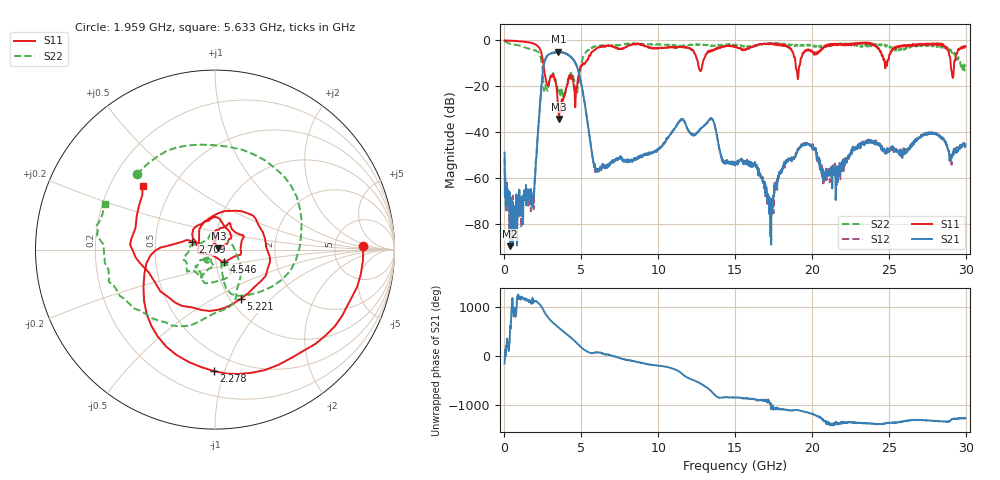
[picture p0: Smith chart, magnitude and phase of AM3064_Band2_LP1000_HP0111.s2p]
# Hz S DB R 50.0
!freq dBS11 angS11 dBS21 angS21 dBS12 angS12 dBS22 angS22
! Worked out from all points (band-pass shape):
!   1600 points, 10 MHz to 29.98 GHz, reference 50 ohm
!   highest |S21| = -4.93 dB at 3.515 GHz (marker M1); lowest = -89.5 dB at 366.1 MHz (marker M2)
!   |S21| within 3 dB of the highest: 2.68 GHz to 4.434 GHz (1.754 GHz wide, 49.3 % of centre)
!   lowest |S11| = -34.2 dB at 3.553 GHz (marker M3), VSWR 1.04, Z = 51.9 + j0.654 ohm
!   |S11| at or under -10 dB: 2.532 GHz to 5.14 GHz (2.608 GHz wide, 68 % of centre); 12.59 GHz to 12.89 GHz (294.3 MHz wide, 2.31 % of centre); 18.93 GHz to 19.24 GHz (302.5 MHz wide, 1.58 % of centre)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
!   |S22| runs from -24.7 to -0.2 dB; largest |S21 - S12| = 0.013
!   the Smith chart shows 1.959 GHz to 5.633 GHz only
!   S11 on the Smith chart (normalised r, x): 1.959 GHz: 10, +1; 2.278 GHz: 0.37, -0.92; 2.709 GHz: 0.77, +0.07; 4.546 GHz: 1.10, -0.15; 5.221 GHz: 1.12, -0.68; 5.633 GHz: 0.34, +0.34
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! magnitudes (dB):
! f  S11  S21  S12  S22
! 10 MHz  0.0  -48.8  -51.2  -0.2
! 366.1 MHz  -0.1  -89.5  -68.5  -1.4
! 1.959 GHz  -1.7  -62.2  -61.7  -4.4
! 2.278 GHz  -3.4  -31.0  -31.0  -5.9
! 2.709 GHz  -17.5  -7.5  -7.5  -20.4
! 3.515 GHz  -30.5  -4.9  -5.0  -22.5
! 3.553 GHz  -34.2  -5.1  -5.0  -21.5
! 4.546 GHz  -21.3  -9.0  -8.9  -17.4
! 5.015 GHz  -11.1  -19.5  -19.5  -9.5
! 5.221 GHz  -10.2  -27.3  -27.2  -5.9
! 5.633 GHz  -5.4  -46.4  -46.5  -3.5
! 6.045 GHz  -3.3  -56.3  -57.0  -2.5
! 10 GHz  -3.4  -47.7  -47.3  -1.8
! 13.43 GHz  -4.7  -33.9  -33.9  -2.4
! 15 GHz  -2.6  -53.9  -54.5  -1.8
! 16.35 GHz  -2.3  -54.9  -53.9  -2.5
! 17.31 GHz  -1.6  -85.4  -71.6  -1.4
! 18.29 GHz  -2.2  -52.6  -52.6  -1.9
! 19.99 GHz  -4.6  -46.0  -45.7  -2.0
! 20.83 GHz  -3.0  -60.7  -58.5  -2.3
! 25 GHz  -8.0  -48.2  -47.2  -2.3
! 29.98 GHz  -2.5  -45.3  -46.3  -10.5
